(* Logix 5000 AddOnInstructionDefinition export ACS_SOFTWARE_STOP; software revision 20.01 *)

ADD_ON_INSTRUCTION ACS_SOFTWARE_STOP   (* revision 2.0, vendor Tolomatic, Inc *)
// Sends a network ESTOP command
VAR_IN_OUT
   DriveCMD : SINT; {required}   // ACS.O.CMD
END_VAR

ROUTINE Logic   (* ladder *)
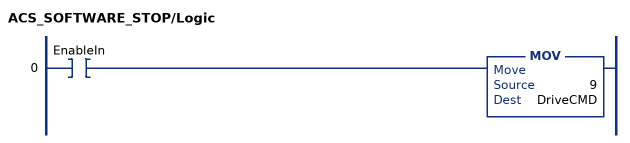
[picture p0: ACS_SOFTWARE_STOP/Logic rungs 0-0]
   0: XIC(EnableIn)MOV(9,DriveCMD);
END_ROUTINE
END_ADD_ON_INSTRUCTION
